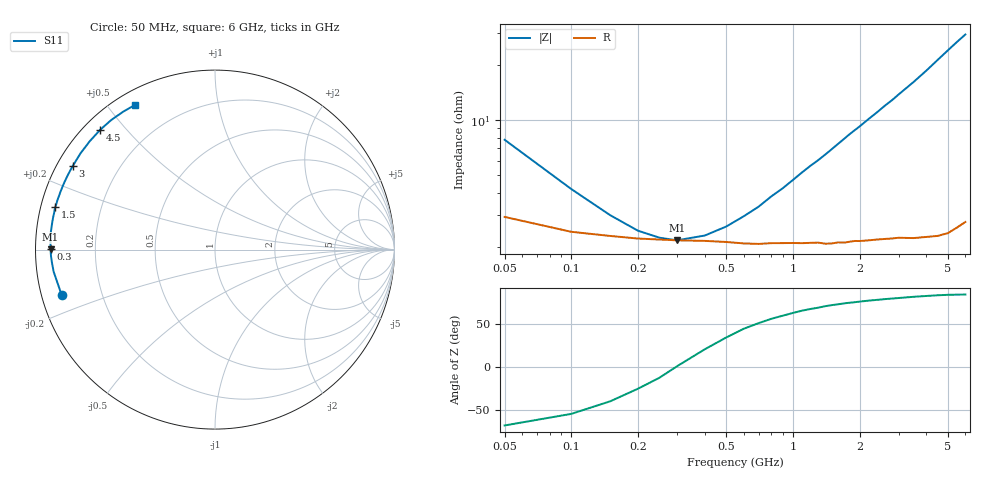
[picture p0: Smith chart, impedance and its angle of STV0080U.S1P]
! SIEMENS Discrete & RF Semiconductors
! BA892
! Si PIN Diode in SCD-80
! IF = 0.08 mA
! S-Parameters:  September  1997
# GHz  S  MA  R  50
!  f  S11
! GHz  MAG  ANG
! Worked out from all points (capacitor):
!   34 points, 50 MHz to 6 GHz, reference 50 ohm
!   read as one part to ground: C = 415 pF near 50 MHz
!   lowest |Z| = 2.19 ohm at 300 MHz (marker M1)
!   series resonance near 295.8 MHz, so ESL is about 700 pH
!   S11 on the Smith chart (normalised r, x): 50 MHz: 0.06, -0.14; 300 MHz: 0.04, +0.00; 1.5 GHz: 0.04, +0.13; 3 GHz: 0.05, +0.27; 4.5 GHz: 0.05, +0.43; 6 GHz: 0.06, +0.59
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0.05  0.891 -163.5
0.1  0.9074 -172.2
0.15  0.9117 -175.6
0.2  0.9143 -177.6
0.3  0.9161 179.9
0.4  0.9167 178.1
0.5  0.9178 176.6
0.6  0.9193 175.2
0.7  0.9199 174.0
0.8  0.9192 172.7
0.9  0.9193 171.6
1.1  0.9196 169.2
1.4  0.9206 166.0
1.5  0.9206 164.9
1.6  0.9197 163.8
1.8  0.9196 161.6
2  0.9193 159.6
2.2  0.9191 157.5
2.4  0.919 155.5
2.6  0.919 153.4
2.8  0.9192 151.5
3  0.9192 149.4
3.5  0.9215 144.4
4  0.9228 139.2
4.5  0.9246 133.8
5  0.925 128.6
5.5  0.9231 123.6
6  0.9212 119.0
